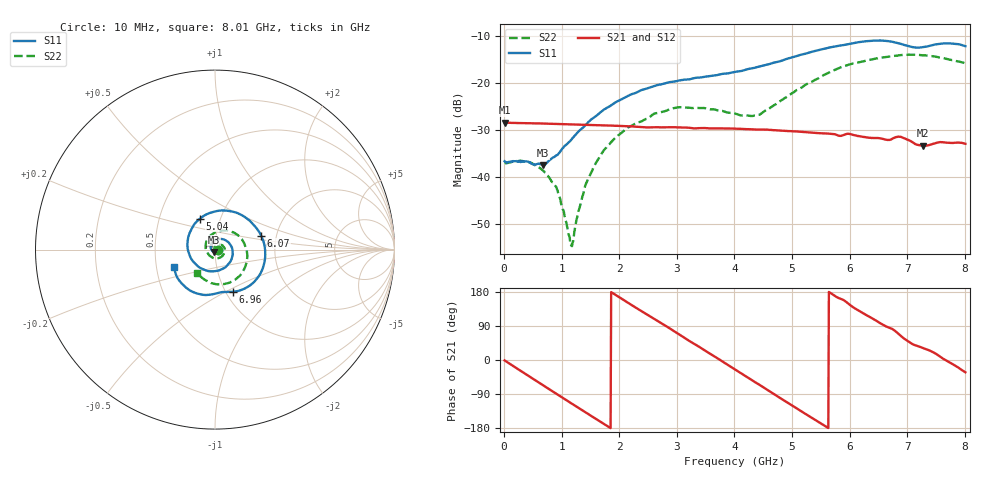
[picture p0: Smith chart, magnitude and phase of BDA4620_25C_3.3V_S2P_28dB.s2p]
!Agilent Technologies,E5071B,MY42404982,A.09.10
!Date: Wed May 06 08:54:54 2026
!Data & Calibration Information:
!Freq	S11:SOLT2(ON)	S21:SOLT2(ON)	S12:SOLT2(ON)	S22:SOLT2(ON)
# Hz S RI R 50
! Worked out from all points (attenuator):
!   801 points, 10 MHz to 8.01 GHz, reference 50 ohm
!   highest |S21| = -28.37 dB at 10 MHz (marker M1); lowest = -33.3 dB at 7.27 GHz (marker M2)
!   lowest |S11| = -37.5 dB at 680 MHz (marker M3), VSWR 1.03, Z = 49.6 - j1.28 ohm
!   |S11| at or under -10 dB: start of sweep to end of sweep
!   |S22| runs from -54.7 to -13.9 dB; largest |S21 - S12| = 0.00021
!   S11 on the Smith chart (normalised r, x): 10 MHz: 1.03, -0.00; 5.04 GHz: 0.80, +0.29; 6.07 GHz: 1.66, +0.28; 6.96 GHz: 1.08, -0.54; 8.01 GHz: 0.62, -0.13
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1e7  0.0148 -0.000945  0.0382 -0.000762  0.0382 -0.000787  0.014 -0.00045
4.2e8  0.00791 -0.0123  0.0282 -0.0249  0.0282 -0.0249  0.0136 -0.00495
6.8e8  -0.00376 -0.0129  0.0146 -0.0343  0.0147 -0.0344  0.0094 -0.00699
9.3e8  -0.0164 -0.0058  -0.000747 -0.0369  -0.000778 -0.037  0.00354 -0.00628
1.16e9  -0.0233 0.00849  -0.0146 -0.0335  -0.0146 -0.0336  -0.00146 -0.00119
1.2e9  -0.0238 0.0116  -0.0168 -0.0324  -0.0168 -0.0324  -0.00207 3.14e-05
1.35e9  -0.0233 0.0234  -0.0242 -0.027  -0.0243 -0.027  -0.00364 0.0046
1.53e9  -0.0169 0.0384  -0.0309 -0.0185  -0.0309 -0.0185  -0.00343 0.0112
1.77e9  0.00131 0.0539  -0.0353 -0.00489  -0.0353 -0.00484  0.000624 0.0205
2.14e9  0.0441 0.0579  -0.0309 0.0162  -0.031 0.0162  0.0164 0.0291
2.68e9  0.0961 0.00488  -0.00699 0.0332  -0.00689 0.0333  0.0443 0.0197
3.08e9  0.0879 -0.0633  0.015 0.0303  0.0151 0.0304  0.0552 -0.00715
4.01e9  -0.09 -0.0971  0.0298 -0.0139  0.0298 -0.0139  -0.0102 -0.0465
4.42e9  -0.1505 -0.00352  0.014 -0.0289  0.0141 -0.029  -0.0444 -0.0129
5.04e9  -0.0834 0.1724  -0.0171 -0.0256  -0.0171 -0.0256  -0.0266 0.0767
5.35e9  0.0197 0.2165  -0.0266 -0.0134  -0.0266 -0.0135  0.0228 0.1018
6.07e9  0.2572 0.0781  -0.0211 0.0186  -0.0211 0.0187  0.1557 0.0481
6.68e9  0.2066 -0.1905  0.00193 0.0248  0.00191 0.0249  0.1703 -0.0899
6.96e9  0.0991 -0.235  0.0147 0.0212  0.0148 0.0212  0.1328 -0.1503
7.27e9  0.016 -0.2423  0.0184 0.0114  0.0185 0.0115  0.0603 -0.1897
7.64e9  -0.1244 -0.2353  0.0235 0.000719  0.0235 0.000783  -0.0309 -0.1825
8.01e9  -0.2278 -0.0991  0.0192 -0.0121  0.0192 -0.0121  -0.1016 -0.1277
